TYPE Warning :
STRUCT
	//PRESSURE_Alarm:BOOL;
	PRESSURE:BOOL;
	
	//MFC1_Alarm:BOOL;
	MFC1:BOOL;
	
	//MFC2_Alarm:BOOL;
	MFC2:BOOL;
	
	//MFC3_Alarm:BOOL;
	MFC3:BOOL;
	
	//MFC4_Alarm:BOOL;
	MFC4:BOOL;
	
	//MFC5_Alarm:BOOL;
	MFC5:BOOL;
	
	//MFC6_Alarm:BOOL;
	MFC6:BOOL;
	
	//MFC7_Alarm:BOOL;
	MFC7:BOOL;
	
	//MFC8_Alarm:BOOL;
	MFC8:BOOL;
	
	//MFC9_Alarm:BOOL;
	MFC9:BOOL;
	
	//WALL_TEMP_Alarm:BOOL;
	WALL_TEMP:BOOL;
	
	//LID_TEMP_Alarm:BOOL;
	LID_TEMP:BOOL;
	
	//STAGE_EDGE_TEMP_Alarm:BOOL;
	STAGE_EDGE_TEMP:BOOL;
	
	//STAGE_CENTER_TEMP_ALARM: BOOL;
	STAGE_CENTER_TEMP: BOOL;
	
	
	CHILLER1:BOOL;
	CHILLER2:BOOL;
	
	
	
	OpenCloseSlitValveTimeout:BOOL;
	Gas1FlowPressureOutOfRange:BOOL;
	Gas2FlowPressureOutOfRange:BOOL;
	Gas3FlowPressureOutOfRange:BOOL;
	Gas4FlowPressureOutOfRange:BOOL;
	Gas5FlowPressureOutOfRange:BOOL;
	Gas6FlowPressureOutOfRange:BOOL;
	Gas7FlowPressureOutOfRange:BOOL;
	Gas8FlowPressureOutOfRange:BOOL;
	Gas9FlowPressureOutOfRange:BOOL;	
	
	
	//PROCESS TOLERANCE
	TOLERANCE_PRESSURE:BOOL;
	TOLERANCE_MFC1:BOOL;
	TOLERANCE_MFC2:BOOL;
	TOLERANCE_MFC3:BOOL;
	TOLERANCE_MFC4:BOOL;
	TOLERANCE_MFC5:BOOL;
	TOLERANCE_MFC6:BOOL;
	TOLERANCE_MFC7:BOOL;
	TOLERANCE_MFC8:BOOL;
	TOLERANCE_MFC9:BOOL;
	TOLERANCE_WALL_TEMP:BOOL;
	TOLERANCE_LID_TEMP:BOOL;
	TOLERANCE_STAGE_EDGE_TEMP:BOOL;
	TOLERANCE_STAGE_CENTER_TEMP: BOOL;	
	

END_STRUCT
END_TYPE
